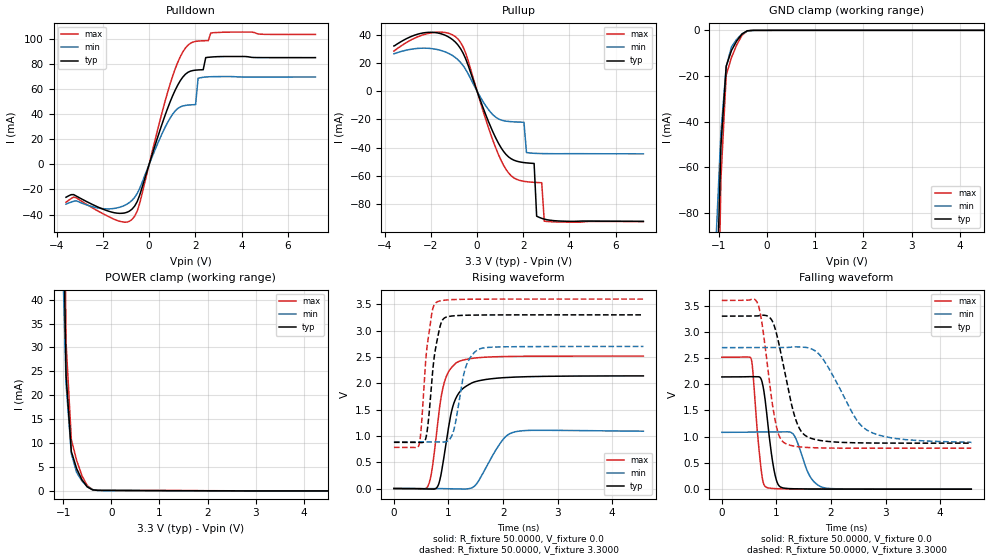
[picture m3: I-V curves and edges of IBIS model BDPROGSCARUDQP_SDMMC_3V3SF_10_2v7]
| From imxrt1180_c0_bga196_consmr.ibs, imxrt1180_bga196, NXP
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[Model]  BDPROGSCARUDQP_SDMMC_3V3SF_10_2v7
|   Model BDPROGSCARUDQP_SDMMC_3V3SF_10_2v7
| This model was characterised for following simulation conditions:
| External (pad) voltage:
|   - Typ: 3.3V,   - Min: 2.7V,   - Max: 3.6V
| Library cells for typ/min/max conditions are connected as defined below:
|  IO - External Pad
|  A - Core Input
|  EN - Output Buffer Enable
|  ASRCN3V3[0] - REFH3V3
|  ASRCN3V3[1] - REFH3V3 REFH3V3 gnde
|  ASRCN3V3[2] - gnde REFH3V3 gnde
|  ASRCN3V3[3] - gnde REFH3V3 gnde
|  ASRCP3V3[0] - vdde3v3 REFL3V3 REFL3V3
|  ASRCP3V3[1] - vdde3v3 REFL3V3 vdde3v3
|  ASRCP3V3[2] - REFL3V3 REFL3V3 vdde3v3
|  ASRCP3V3[3] - REFL3V3 REFL3V3 vdde3v3
|  IOGC - NC
|  PDRV - gnd
|  PSW - vdd
|  REFH3V3 - REFH3V3
|  REFL3V3 - REFL3V3
|  ZI - NC
|  gnd - gnd
|  gnde - gnde
|  vdd - vdd
|  vdde3v3 - vdde3v3
| All other pins connected to ground
Model_type I/O
Polarity   Non-Inverting
Enable   Active-Low
Vinl =   0.6750V
Vinh =   2.2500V
Vmeas =  1.6500V
Cref =   30.0000pF
Rref =   1.0000M
Vref =   3.3000V
C_comp   2.1236pF   2.1010pF   2.1446pF
|C_comp_pullup   0.3619pF   0.3769pF   0.3519pF
|C_comp_pulldown   0.6265pF   0.6593pF   0.5997pF
[Model Spec]
| variable   typ   min   max
Vinh   2.0625V   1.6875V   2.2500V
Vinl   0.8250V   0.6750V   0.9000V
[Temperature Range]   25.0000   0.1050k   -20.0000
[Voltage Range]   3.3000V   2.7000V   3.6000V
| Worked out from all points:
|   slope of the pulldown table from 0 to 0.495 V, typ, clamps not added: 17.2 ohm
|   slope of the pullup table from 0 to 0.495 V, typ, clamps not added: 23 ohm
|   GND clamp passes 1 mA (typ) near -0.48 V on its own axis
|   POWER clamp passes 1 mA (typ) near -0.51 V on its own axis
|   rising waveform, R_fixture 50.0000, V_fixture 0.0: 20-80 % time 243ps typ, 363ps min, 205ps max; typ from 0 V to 2.14 V
|   rising waveform, R_fixture 50.0000, V_fixture 3.3000: 20-80 % time 152ps typ, 198ps min, 140ps max; typ from 0.878 V to 3.3 V
|   falling waveform, R_fixture 50.0000, V_fixture 0.0: 20-80 % time 153ps typ, 237ps min, 120ps max; typ from 2.14 V to 0 V
|   falling waveform, R_fixture 50.0000, V_fixture 3.3000: 20-80 % time 307ps typ, 576ps min, 217ps max; typ from 3.3 V to 0.877 V
[Pulldown]
|Voltage   I(typ)   I(min)   I(max)
-3.6V     -26.23mA   -31.7mA    -30.21mA
-3.16V    -25.23mA   -29.01mA   -26.61mA
-1.4V     -38.9mA    -34.77mA   -44.66mA
-630mV    -33.34mA   -26.4mA    -41.42mA
1.02V     54.81mA    40.1mA     70.52mA
1.79V     74.36mA    47.44mA    96.61mA
2.01V     75.15mA    47.66mA    98.09mA
2.12V     75.31mA    68.67mA    98.35mA
2.34V     75.48mA    69.44mA    98.57mA
2.56V     85.39mA    69.82mA    98.66mA
2.78V     85.72mA    69.96mA    105mA
7.2V      85.14mA    69.68mA    103.6mA
[Pullup]
|Voltage   I(typ)   I(min)   I(max)
-3.6V     31.94mA    26.42mA    28.32mA
-2.04V    41.59mA    30.2mA     41.02mA
-830mV    32.67mA    22.24mA    36.89mA
490mV     -21.3mA    -12.95mA   -25.62mA
1.15V     -42.62mA   -20.86mA   -52.41mA
2.03V     -50.44mA   -21.95mA   -63.68mA
2.14V     -50.64mA   -43.35mA   -63.92mA
2.47V     -51.06mA   -43.88mA   -64.39mA
2.58V     -88.31mA   -43.96mA   -64.49mA
2.8V      -89.83mA   -44.07mA   -64.67mA
2.91V     -90.37mA   -44.1mA    -91.82mA
7.2V      -91.99mA   -44.27mA   -92.07mA
[GND_clamp]
|Voltage   I(typ)   I(min)   I(max)
-3.6V     -5.131A    -2.966A    -8.406A
-1.07V    -134.2mA   -96.06mA   -200.7mA
-960mV    -50.84mA   -45.02mA   -65.28mA
-850mV    -15.74mA   -15.88mA   -19.63mA
-740mV    -8.808mA   -7.25mA    -11.89mA
-630mV    -4.596mA   -3.893mA   -6.316mA
-520mV    -1.551mA   -1.564mA   -2.126mA
-410mV    -182.3uA   -311.4uA   -219.4uA
-190mV    -16.94uA   -12.12uA   -23.77uA
7.2V      0A         0A         0A
[POWER_clamp]
|Voltage   I(typ)   I(min)   I(max)
-3.6V     5.01A      2.849A     8.324A
-1.05V    90.64mA    63.65mA    144.9mA
-940mV    24.29mA    22.45mA    31.15mA
-830mV    8.246mA    7.775mA    10.76mA
-720mV    4.663mA    3.883mA    6.37mA
-610mV    2.344mA    2.086mA    3.186mA
-500mV    850.8uA    898.3uA    1.111mA
-390mV    222uA      282.9uA    270.2uA
-170mV    103uA      69.45uA    142.4uA
7.2V      0A         0A         0A
[Ramp]
| variable   typ   min   max
dV/dt_r  1.2834/0.2433n   0.6535/0.3634n   1.5089/0.2048n
dV/dt_f  1.4527/0.3068n   1.0820/0.5758n   1.6899/0.2167n
R_load = 50.0000
[Rising Waveform]
R_fixture= 50.0000
V_fixture= 0.0
V_fixture_min= 0.0
V_fixture_max= 0.0
|time   V(typ)   V(min)   V(max)
0s        133.3uV    97uV       163.4uV
629ps     -10.2mV    141uV      58.43mV
702.1ps   -11mV      140.8uV    387.4mV
797.3ps   33.12mV    -34.18uV   1.196V
895ps     457mV      -2.004mV   1.898V
1.043ns   1.405V     -6.198mV   2.282V
1.159ns   1.763V     -6.263mV   2.398V
1.482ns   2.027V     51.51mV    2.478V
2.194ns   2.116V     1.07V      2.51V
4.57ns    2.139V     1.089V     2.515V
[Rising Waveform]
R_fixture= 50.0000
V_fixture= 3.3000
V_fixture_min= 2.7000
V_fixture_max= 3.6000
|time   V(typ)   V(min)   V(max)
0s        877.7mV    886.3mV    782.1mV
459.3ps   876.7mV    886.4mV    825.5mV
599.5ps   1.03V      886.4mV    2.624V
701.9ps   2.138V     886.4mV    3.369V
780.9ps   2.762V     886.2mV    3.539V
884.5ps   3.191V     882.5mV    3.571V
1.064ns   3.277V     1.012V     3.588V
1.314ns   3.291V     2.304V     3.595V
1.56ns    3.296V     2.647V     3.597V
4.57ns    3.299V     2.699V     3.598V
[Falling Waveform]
R_fixture= 50.0000
V_fixture= 0.0
V_fixture_min= 0.0
V_fixture_max= 0.0
|time   V(typ)   V(min)   V(max)
0s        2.139V     1.084V     2.515V
538.9ps   2.145V     1.089V     2.479V
710.2ps   2.118V     1.091V     459.5mV
813.8ps   1.524V     1.091V     36.38mV
960.2ps   343.7mV    1.091V     11.23mV
1.099ns   29.89mV    1.092V     6.201mV
1.319ns   7.533mV    1.035V     2.905mV
1.596ns   3.344mV    279mV      1.221mV
1.844ns   1.777mV    35.18mV    623.2uV
4.57ns    133.5uV    172uV      163.4uV
[Falling Waveform]
R_fixture= 50.0000
V_fixture= 3.3000
V_fixture_min= 2.7000
V_fixture_max= 3.6000
|time   V(typ)   V(min)   V(max)
0s        3.299V     2.699V     3.598V
658.7ps   3.303V     2.699V     3.535V
743ps     3.317V     2.699V     3.115V
977.7ps   3.056V     2.7V       1.306V
1.154ns   2.225V     2.7V       877.1mV
1.368ns   1.284V     2.714V     813.3mV
1.613ns   977.4mV    2.685V     792.6mV
1.855ns   919.8mV    2.476V     785.1mV
2.684ns   880.2mV    1.111V     780.9mV
4.57ns    877.3mV    895.4mV    781.8mV
